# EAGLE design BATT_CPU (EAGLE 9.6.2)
COMPANY: ADAFRUIT INDUSTRIES; DRAWN: KTOWN; REV: B
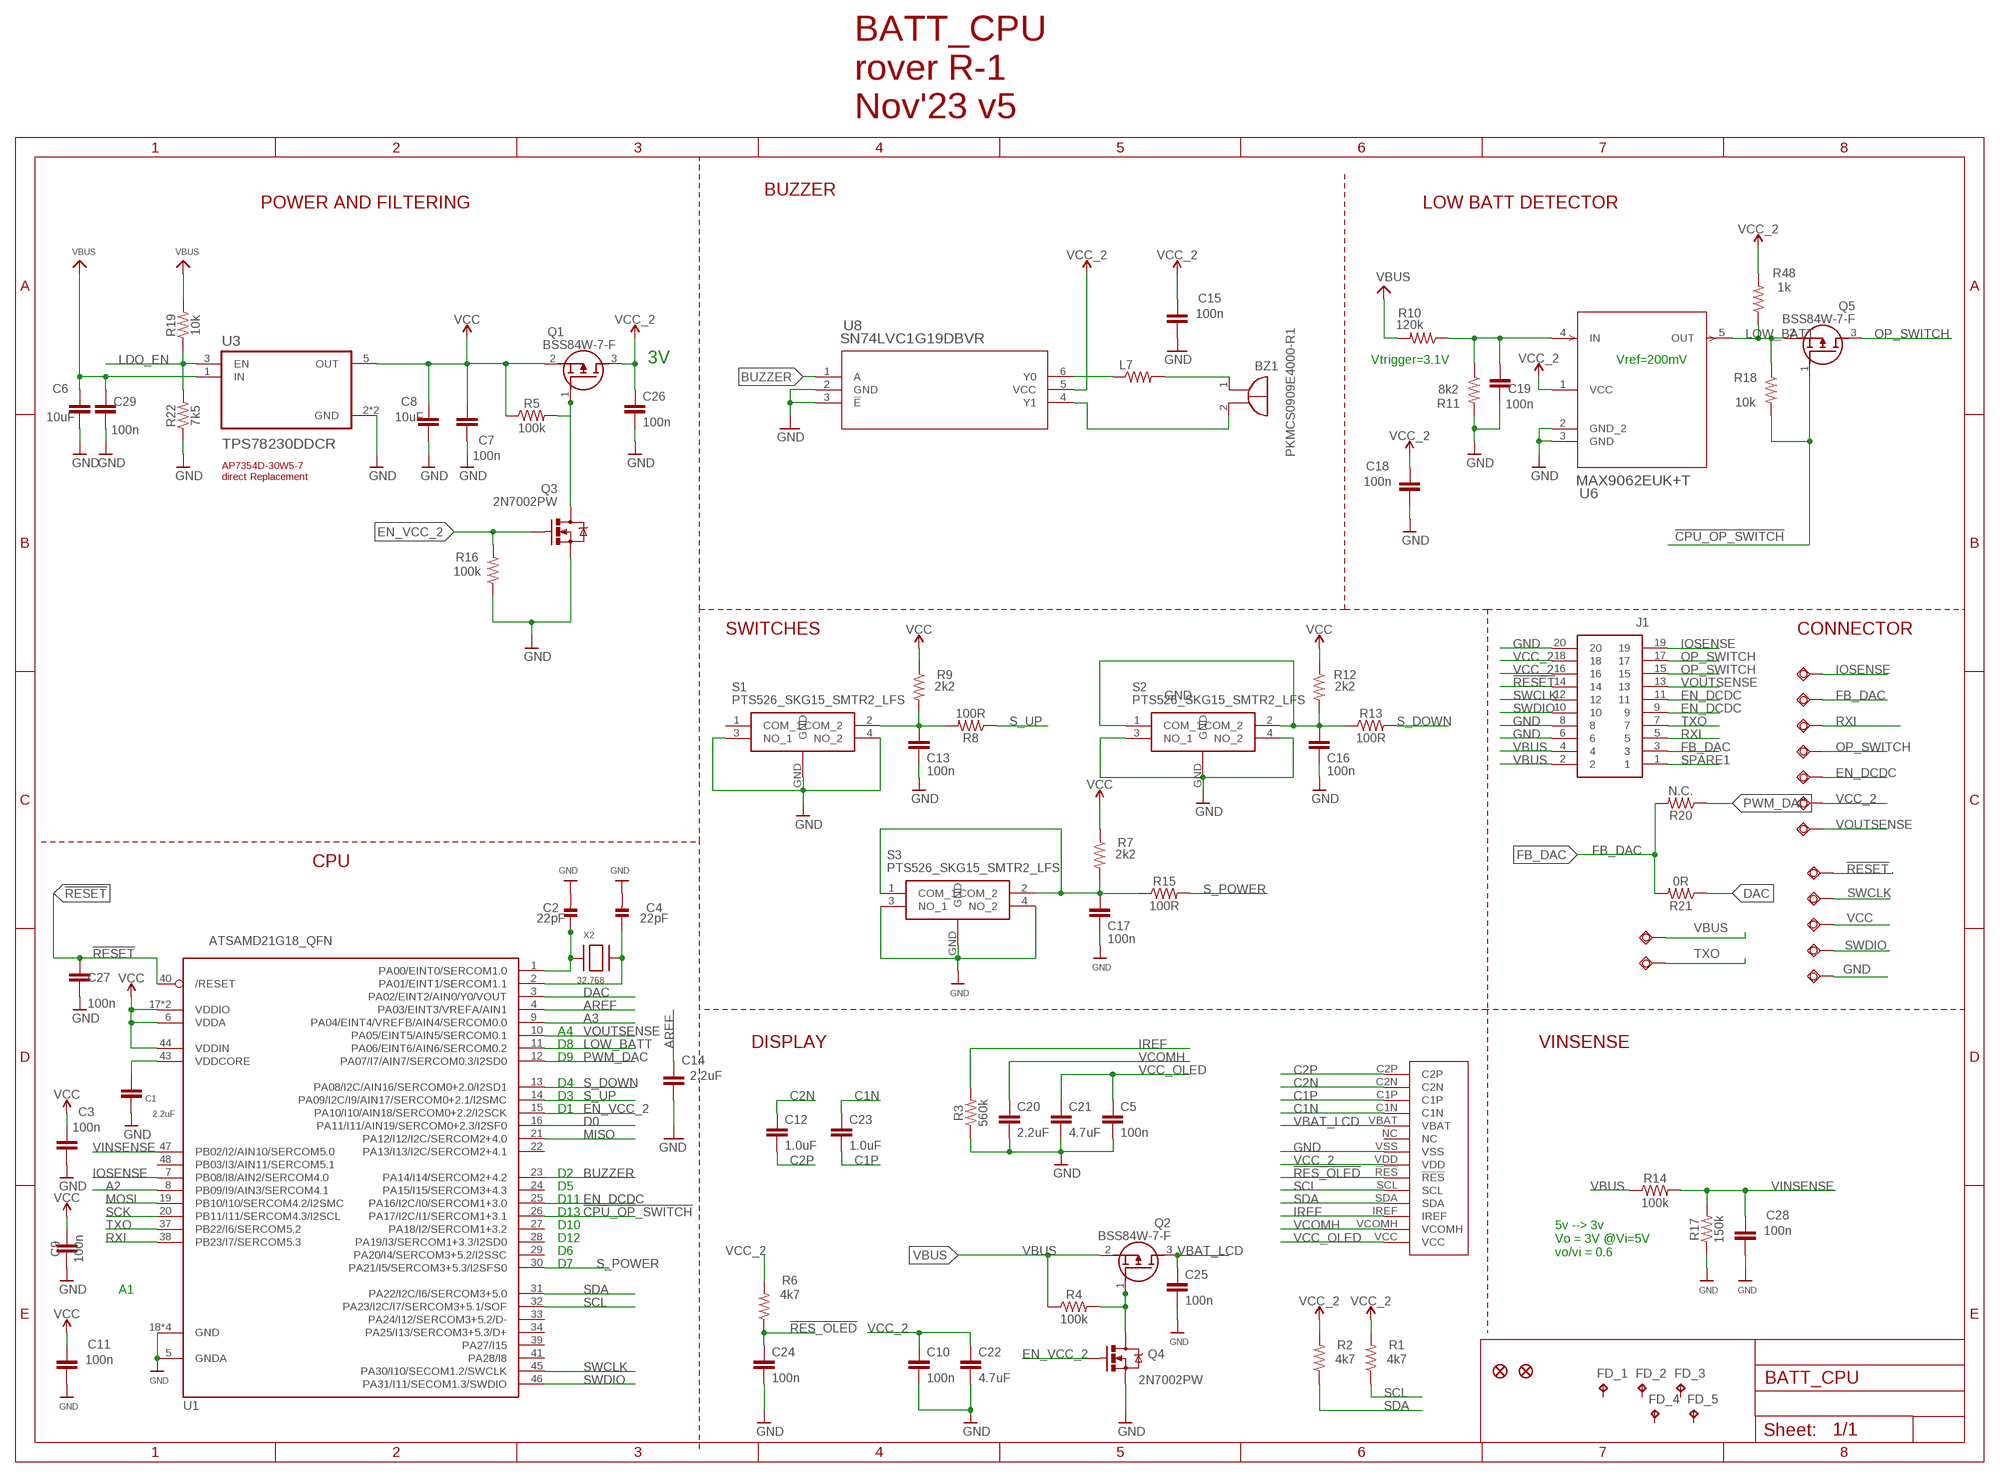
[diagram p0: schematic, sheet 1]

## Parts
BZ1  PKMCS0909E4000-R1  [PKMCS0909]
C1  2.2uF  2.2UF-0603-10V-20%  [0603]
C2  22pF  CAP_CERAMIC0603_NO  [0603-NO]
C3  100n  0.1UF-0402-16V-10%  [0402]
C4  22pF  CAP_CERAMIC0603_NO  [0603-NO]
C5  100n  0.1UF-0402-16V-10%  [0402]
C6  10uF  2.2UF-0603-10V-20%  [0603]
C7  100n  0.1UF-0402-16V-10%  [0402]
C8  10uF  2.2UF-0603-10V-20%  [0603]
C9  100n  0.1UF-0402-16V-10%  [0402]
C10  100n  0.1UF-0402-16V-10%  [0402]
C11  100n  0.1UF-0402-16V-10%  [0402]
C12  1.0uF  1.0UF-0402-16V-10%  [0402]
C13  100n  0.1UF-0402-16V-10%  [0402]
C14  2.2uF  2.2UF-0603-10V-20%  [0603]
C15  100n  0.1UF-0402-16V-10%  [0402]
C16  100n  0.1UF-0402-16V-10%  [0402]
C17  100n  0.1UF-0402-16V-10%  [0402]
C18  100n  0.1UF-0402-16V-10%  [0402]
C19  100n  0.1UF-0402-16V-10%  [0402]
C20  2.2uF  2.2UF-0603-10V-20%  [0603]
C21  4.7uF  4.7UF0603  [0603]
C22  4.7uF  4.7UF0603  [0603]
C23  1.0uF  1.0UF-0402-16V-10%  [0402]
C24  100n  0.1UF-0402-16V-10%  [0402]
C25  100n  0.1UF-0402-16V-10%  [0402]
C26  100n  0.1UF-0402-16V-10%  [0402]
C27  100n  0.1UF-0402-16V-10%  [0402]
C28  100n  0.1UF-0402-16V-10%  [0402]
C29  100n  0.1UF-0402-16V-10%  [0402]
EN_DCDC  TESTPAD_TPSQB1,27  [TESTPAD_B1,27]
FB_DAC  TESTPAD_TPSQB1,27  [TESTPAD_B1,27]
FD_1  FD_1  TPTP06SQ  [TP06SQ]
FD_2  FD_1  TPTP06SQ  [TP06SQ]
FD_3  FD_1  TPTP06SQ  [TP06SQ]
FD_4  FD_1  TPTP06SQ  [TP06SQ]
FD_5  FD_1  TPTP06SQ  [TP06SQ]
IOSENSE  TESTPAD_TPSQB1,27  [TESTPAD_B1,27]
J1  DF40C_2.0_-20DS-0.4V_51_  [DF40C2020DS04V51]
L7  MMZ2012Y202BT000  RESISTOR0805-RES  [0805]
OP_SWITCH  TESTPAD_TPSQB1,27  [TESTPAD_B1,27]
Q1  BSS84W-7-F  [SOT65P222X110-3N]
Q2  BSS84W-7-F  [SOT65P222X110-3N]
Q3  2N7002PW  MOSFET-NCHANNEL2N7002PW  [SOT323]
Q4  2N7002PW  MOSFET-NCHANNEL2N7002PW  [SOT323]
Q5  BSS84W-7-F  [SOT65P222X110-3N]
R1  4k7  RESISTOR0402  [0402]
R2  4k7  RESISTOR0402  [0402]
R3  560k  RESISTOR0402  [0402]
R4  100k  RESISTOR0402  [0402]
R5  100k  RESISTOR0402  [0402]
R6  4k7  RESISTOR0402  [0402]
R7  2k2  RESISTOR0402  [0402]
R8  100R  RESISTOR0402  [0402]
R9  2k2  RESISTOR0402  [0402]
R10  120k  RESISTOR0402  [0402]
R11  8k2  RESISTOR0402  [0402]
R12  2k2  RESISTOR0402  [0402]
R13  100R  RESISTOR0402  [0402]
R14  100k  RESISTOR0402  [0402]
R15  100R  RESISTOR0402  [0402]
R16  100k  RESISTOR0402  [0402]
R17  150k  RESISTOR0402  [0402]
R18  10k  RESISTOR0402  [0402]
R19  10k  RESISTOR0402  [0402]
R20  N.C.  RESISTOR0402  [0402]
R21  0R  RESISTOR0402  [0402]
R22  7k5  RESISTOR0402  [0402]
R48  1k  RESISTOR0402  [0402]
RXI  TESTPAD_TPSQB1,27  [TESTPAD_B1,27]
S1  PTS526_SKG15_SMTR2_LFS  [PTS526SKG15SMTR2LFS]
S2  PTS526_SKG15_SMTR2_LFS  [PTS526SKG15SMTR2LFS]
S3  PTS526_SKG15_SMTR2_LFS  [PTS526SKG15SMTR2LFS]
U1  ATSAMD21G18_QFN  ATSAMD21J_QFN  [TQFN48_7MM]
U3  TPS78230DDCR  [SOT95P280X110-5N]
U6  MAX9062EUK+T  [21-0057F_MXM]
U8  SN74LVC1G19DBVR  [DBV6]
U$30  64X32_OLED_049  [LCD_14_PINS]
U$34  FIDUCIAL""  [FIDUCIAL_1MM]
U$35  FIDUCIAL""  [FIDUCIAL_1MM]
VBUS  TESTPAD_TPSQB1,27  [TESTPAD_B1,27]
VBUS1  TESTPAD_TPSQB1,27  [TESTPAD_B1,27]
VBUS2  TESTPAD_TPSQB1,27  [TESTPAD_B1,27]
VBUS3  TESTPAD_TPSQB1,27  [TESTPAD_B1,27]
VBUS4  TESTPAD_TPSQB1,27  [TESTPAD_B1,27]
VBUS5  TESTPAD_TPSQB1,27  [TESTPAD_B1,27]
VBUS6  TESTPAD_TPSQB1,27  [TESTPAD_B1,27]
VCC_2  TESTPAD_TPSQB1,27  [TESTPAD_B1,27]
VOUTSENSE  TESTPAD_TPSQB1,27  [TESTPAD_B1,27]
X2  32.768  XTAL-3.2X1.5  [XTAL3215]

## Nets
!CPU_OP_SWITCH: Q5.1(G) R18.2 U1.26(PA17/I2C/I1/SERCOM1+3.1)
!RES_OLED: C24.1 R6.1 U$30.!RES
!RESET: C27.1 J1.14 U1.40(/RESET) VBUS1.TP
A2: U1.8(PB09/I9/AIN3/SERCOM4.1)
A3: U1.9(PA04/EINT4/VREFB/AIN4/SERCOM0.0)
AREF: C14.1 U1.4(PA03/EINT3/VREFA/AIN1)
BUZZER: U1.23(PA14/I14/SERCOM2+4.2) U8.1(A)
C1N: C23.1 U$30.C1N
C1P: C23.2 U$30.C1P
C2N: C12.1 U$30.C2N
C2P: C12.2 U$30.C2P
D0: U1.16(PA11/I11/AIN19/SERCOM0+2.3/I2SF0)
DAC: R21.1 U1.3(PA02/EINT2/AIN0/Y0/VOUT)
EN_DCDC: EN_DCDC.TP J1.9 J1.11 U1.25(PA16/I2C/I0/SERCOM1+3.0)
EN_VCC_2: Q3.1(G) Q4.1(G) R16.2 U1.15(PA10/I10/AIN18/SERCOM0+2.2/I2SCK)
FB_DAC: FB_DAC.TP J1.3 R20.2 R21.2
GND: C1.2 C2.2 C3.2 C4.2 C5.2 C6.2 C7.2 C8.2 C9.2 C10.2 C11.2 C13.2 C14.2 C15.2 C16.2 C17.2 C18.2 C19.2 C20.2 C21.2 C22.2 C24.2 C25.2 C26.2 C27.2 C28.2 C29.2 J1.6 J1.8 J1.20 Q3.2(S) Q4.2(S) R3.1 R11.2 R16.1 R17.1 R22.1 S1.3(NO_1) S1.4(NO_2) S1.GND S2.3(NO_1) S2.4(NO_2) S2.GND S3.3(NO_1) S3.4(NO_2) S3.GND U1.5(GNDA) U1.18(GND) U1.35(GND) U1.42(GND) U1.THERMAL(GND) U3.2(GND) U3.4(GND) U6.2(GND_2) U6.3(GND) U8.2(GND) U8.3(!E) U$30.VSS VBUS4.TP
IOSENSE: IOSENSE.TP J1.19 U1.7(PB08/I8/AIN2/SERCOM4.0)
IREF: R3.2 U$30.IREF
LDO_EN: R19.1 R22.2 U3.3(EN)
LOW_BATT: Q5.2(S) R18.1 R48.1 U1.11(PA06/EINT6/AIN6/SERCOM0.2) U6.5(OUT)
MISO: U1.21(PA12/I12/I2C/SERCOM2+4.0)
MOSI: U1.19(PB10/I10/SERCOM4.2/I2SMC)
N$1: C17.1 R7.2 R15.1 S3.1(COM_1) S3.2(COM_2)
N$2: C13.1 R8.2 R9.2 S1.2(COM_2)
N$3: C16.1 R12.2 R13.1 S2.1(COM_1) S2.2(COM_2)
N$4: Q2.1(G) Q4.3(D) R4.2
N$5: C2.1 U1.1(PA00/EINT0/SERCOM1.0) X2.P$1
N$6: Q1.1(G) Q3.3(D) R5.2
N$7: C4.1 U1.2(PA01/EINT1/SERCOM1.1) X2.P$2
N$10: C19.1 R10.1 R11.1 U6.4(IN)
N$17: L7.1 U8.6(Y0)
N$19: BZ1.1(+) L7.2
N$22: BZ1.2(-) U8.4(Y1)
OP_SWITCH: J1.15 J1.17 OP_SWITCH.TP Q5.3(D)
PWM_DAC: R20.1 U1.12(PA07/I7/AIN7/SERCOM0.3/I2SD0)
RXI: J1.5 RXI.TP U1.38(PB23/I7/SERCOM5.3)
S_DOWN: R13.2 U1.13(PA08/I2C/AIN16/SERCOM0+2.0/I2SD1)
S_POWER: R15.2 U1.30(PA21/I5/SERCOM3+5.3/I2SFS0)
S_UP: R8.1 U1.14(PA09/I2C/I9/AIN17/SERCOM0+2.1/I2SMC)
SCK: U1.20(PB11/I11/SERCOM4.3/I2SCL)
SCL: R1.1 U1.32(PA23/I2C/I7/SERCOM3+5.1/SOF) U$30.SCL
SDA: R2.1 U1.31(PA22/I2C/I6/SERCOM3+5.0) U$30.SDA
SPARE1: J1.1
SWCLK: J1.12 U1.45(PA30/I10/SECOM1.2/SWCLK) VBUS2.TP
SWDIO: J1.10 U1.46(PA31/I11/SECOM1.3/SWDIO) VBUS3.TP
TXO: J1.7 U1.37(PB22/I6/SERCOM5.2) VBUS6.TP
VBAT_LCD: C25.1 Q2.3(D) U$30.VBAT
VBUS: C6.1 C29.1 J1.2 J1.4 Q2.2(S) R4.1 R10.2 R14.1 R19.2 U3.1(IN) VBUS5.TP
VCC: C3.1 C7.1 C8.1 C9.1 C11.1 Q1.2(S) R5.1 R7.1 R9.1 R12.1 R48.2 U1.6(VDDA) U1.17(VDDIO) U1.36(VDDIO) U1.44(VDDIN) U3.5(OUT) VBUS.TP ; supply symbol labelled VCC_2
VCC_2: C10.1 C15.1 C18.1 C22.1 C26.1 J1.16 J1.18 Q1.3(D) R1.2 R2.2 R6.2 U6.1(VCC) U8.5(VCC) U$30.VDD VCC_2.TP
VCC_OLED: C5.1 C21.1 U$30.VCC
VCOMH: C20.1 U$30.VCOMH
VDDCORE: C1.1 U1.43(VDDCORE)
VINSENSE: C28.1 R14.2 R17.2 U1.47(PB02/I2/AIN10/SERCOM5.0)
VOUTSENSE: J1.13 U1.10(PA05/EINT5/AIN5/SERCOM0.1) VOUTSENSE.TP
Unconnected: FD_1.TP FD_2.TP FD_3.TP FD_4.TP FD_5.TP S1.1(COM_1) U1.22(PA13/I13/I2C/SERCOM2+4.1) U1.24(PA15/I15/SERCOM3+4.3) U1.27(PA18/I2/SERCOM1+3.2) U1.28(PA19/I3/SERCOM1+3.3/I2SD0) U1.29(PA20/I4/SERCOM3+5.2/I2SSC) U1.33(PA24/I12/SERCOM3+5.2/D-) U1.34(PA25/I13/SERCOM3+5.3/D+) U1.39(PA27/I15) U1.41(PA28/I8) U1.48(PB03/I3/AIN11/SERCOM5.1) U$30.NC

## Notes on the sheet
- BATT_CPU
  rover R-1
  Nov'23 v5
- BUZZER
- POWER AND FILTERING | LOW BATT DETECTOR
- 3V | Vtrigger=3.1V | Vref=200mV
- AP7354D-30W5-7 
  direct Replacement
- SWITCHES | CONNECTOR
- CPU
- A4
- D8 | DISPLAY | VINSENSE
- D9
- D4
- D3
- D1
- D2
- D5
- D11
- D13
- D10
- D12
- D6
- D7
- 5v --> 3v
  Vo = 3V @Vi=5V
  vo/vi = 0.6
- A1

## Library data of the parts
BZ1 = buzzer:PKMCS0909E4000-R1: PKMCS0909E4000-R1
C1 C14 C20 = SparkFun-Capacitors:2.2UF: 2.2µF ceramic capacitors; PROD_ID: CAP-07888
C2 C4 = microbuilder:CAP_CERAMIC: Ceramic Capacitors
C3 C5 C7 C9-C11 C13 C15-C19 C24-C29 = SparkFun-Capacitors:0.1UF: 0.1µF ceramic capacitors; PROD_ID: CAP-12416; VALUE: 0.1uF
C6 C8 = SparkFun-Capacitors:2.2UF: 2.2µF ceramic capacitors; PROD_ID: CAP-07888; VALUE: 2.2uF
C12 C23 = SparkFun-Capacitors:1.0UF: 1µF ceramic capacitors; PROD_ID: CAP-12417
C21 C22 = SparkFun-Capacitors:4.7UF: 4.7µF ceramic capacitors; PROD_ID: CAP-08280
EN_DCDC FB_DAC IOSENSE OP_SWITCH RXI VBUS VBUS1-VBUS6 VCC_2 VOUTSENSE = BeagleBone_Blue_R3:TESTPAD_TPSQ: Test pad
FD_1-FD_5 = testpad:TP: Test pad
J1 = DF40C_2.0_-20DS-0.4V_51_:DF40C_2.0_-20DS-0.4V_51_: Board to Board & Mezzanine Connectors 20P 2-ROW RECEPT VERT SMT 2.0MM HGHT Source: Datasheet; DESCRIPTION: Board to Board & Mezzanine Connectors 20P 2-ROW RECEPT VERT SMT 2.0MM HGHT; HEIGHT: 2.1mm; MANUFACTURER_NAME: Hirose; MANUFACTURER_PART_NUMBER: DF40C(2.0)-20DS-0.4V(51); MOUSER_PART_NUMBER: 798-DF40C2020DS04V51; MOUSER_PRICE-STOCK: https://www.mouser.co.uk/ProductDetail/Hirose-Connector/DF40C2.0-20DS-0.4V51?qs=3aug5cyrIbdA5dYbMRd5pw%3D%3D
L7 = SparkFun:RESISTOR: Resistor
Q1 Q2 Q5 = BSS84W-7-F:BSS84W-7-F: Lattice Source: Datasheet; DESCRIPTION: Lattice; HEIGHT: 1.1mm; MANUFACTURER_NAME: Lattice Semiconductor; MANUFACTURER_PART_NUMBER: BSS84W-7-F; MOUSER_PART_NUMBER: N/A; MOUSER_PRICE-STOCK: https://www.mouser.com/Search/Refine.aspx?Keyword=N%2FA
Q3 Q4 = SparkFun-DiscreteSemi:MOSFET-NCHANNEL: Common NMOSFET Parts MFG P/NStore IDProd ID FDD8780TRANS-09984 SI7820DNTRANS-11055 FDS6630AIC-08089 2N7002PWTRANS-11151 FQP30N06L COM-10213TRANS-10060 BSS123LT1GTRANS-08345 BSS138TRANS-00830 BS170 2N7000; PROD_ID: TRANS-11151
R1-R22 R48 = SparkFun-Resistors:RESISTOR: Generic Resistor Package
S1-S3 = PTS526_SKG15_SMTR2_LFS:PTS526_SKG15_SMTR2_LFS: Tact 5.2 x 5.2, 1.5 mm H, 260gf, G leads, Ground pin, metal actuator Source: Datasheet; ARROW_PART_NUMBER: PTS526 SKG15 SMTR2 LFS; ARROW_PRICE-STOCK: https://www.arrow.com/en/products/pts526-skg15-smtr2-lfs/ck?region=nac; DESCRIPTION: Tact 5.2 x 5.2, 1.5 mm H, 260gf, G leads, Ground pin, metal actuator; HEIGHT: 1.6mm; MANUFACTURER_NAME: C & K COMPONENTS; MANUFACTURER_PART_NUMBER: PTS526 SKG15 SMTR2 LFS; MOUSER_PART_NUMBER: 611-PTS526SKG15SMR2L; MOUSER_PRICE-STOCK: https://www.mouser.co.uk/ProductDetail/CK/PTS526-SKG15-SMTR2-LFS?qs=UXgszm6BlbEc7nn5s4cd2Q%3D%3D
U1 = microbuilder:ATSAMD21J
U3 = TPS78230DDCR:TPS78230DDCR: Check prices; AVAILABILITY: Good; DESCRIPTION: 150-mA, nano-IQ, low-dropout voltage regulator with enable from -40C to +125C 5-SOT-23-THIN -40 to 125; MF: Texas Instruments; MP: TPS78230DDCR; PACKAGE: SOT-23-THN-5 Texas Instruments; PRICE: None; PURCHASE-URL: https://pricing.snapeda.com/search/part/TPS78230DDCR/?ref=eda
U6 = MAX9062:MAX9062EUK+T; BUILT_BY: EMA_UL_Team; MANUFACTURER_PART_NUMBER: MAX9062EUK+T; SOURCELIBRARY: Maxim_2014-06-20; VENDOR: Maxim Integrated Products
U8 = SN74LVC1G19DBVR:SN74LVC1G19DBVR; DATASHEET_URL: http://www.ti.com/lit/gpn/SN74LVC1G19; DESCRIPTION: 1-of-2 Decoder/Demultiplexer; FAMILY_NAME: LL Decoder, Mux/Demux; GENERIC_PART_NUMBER: SN74LVC1G19; INDUSTRY_STD_PKG_TYPE: SOT-23; MANUFACTURER: Texas Instruments; MANUFACTURER_PART_NUMBER: SN74LVC1G19DBVR; PACKAGE_DESIGNATOR: DBV; PIN_COUNT: 6; VENDOR: Texas Instruments
U$30 = OLED 66 64x48:64X32_OLED_049
U$34 U$35 = microbuilder:FIDUCIAL: Fiducial Alignment Points; BOM: EXCLUDE
X2 = adafruit2:XTAL: Low cost SMT crystals, no capacitors included

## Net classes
2 gnd: width 0.305 mm, drill 0.483 mm, clearance 0.203 mm

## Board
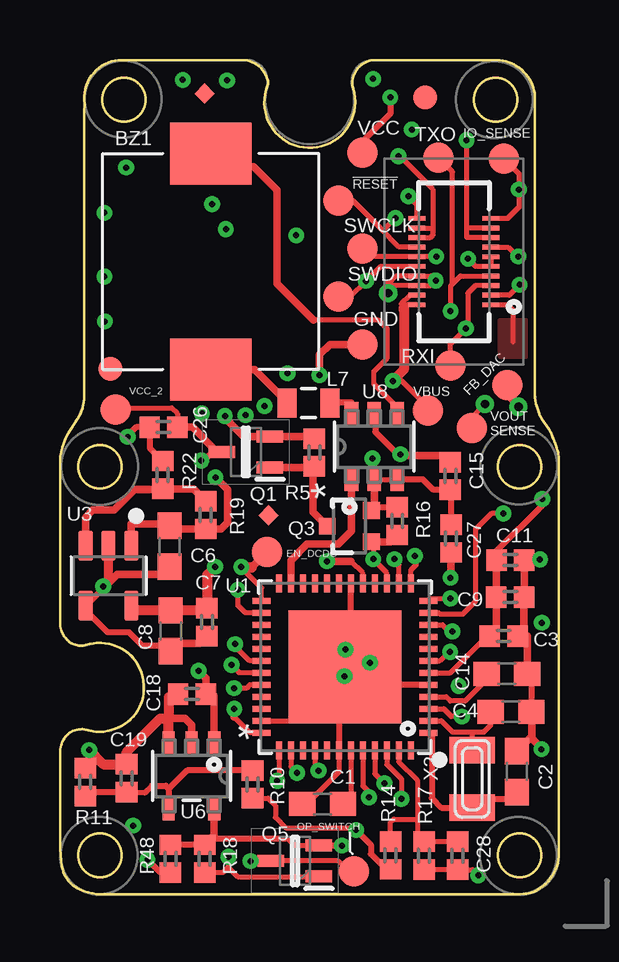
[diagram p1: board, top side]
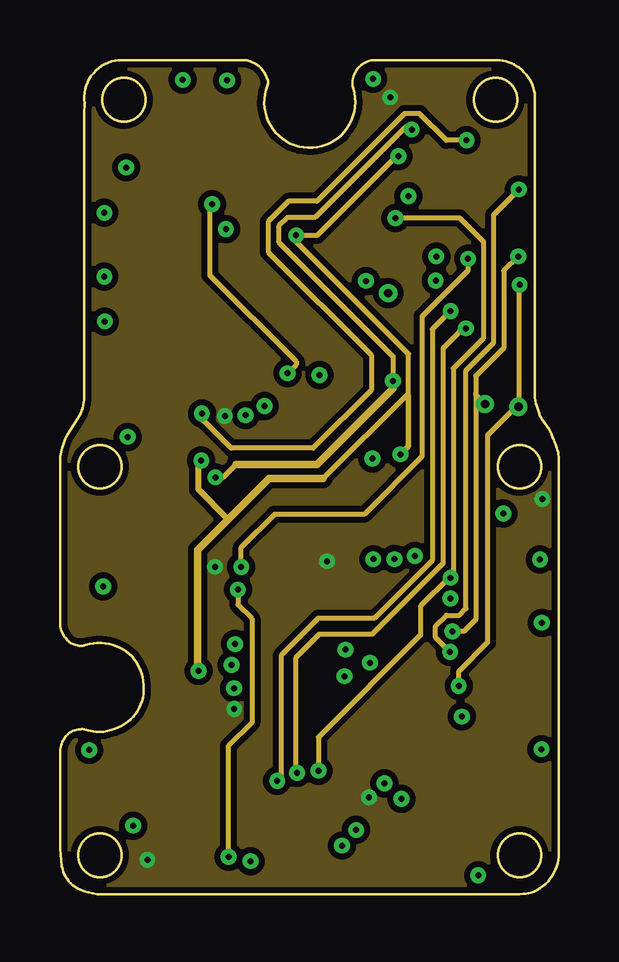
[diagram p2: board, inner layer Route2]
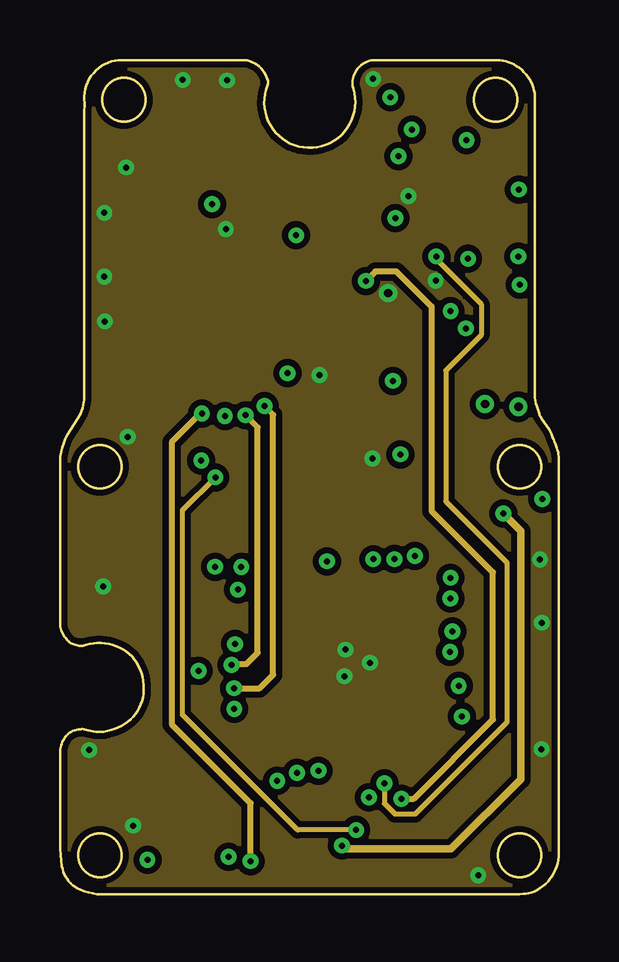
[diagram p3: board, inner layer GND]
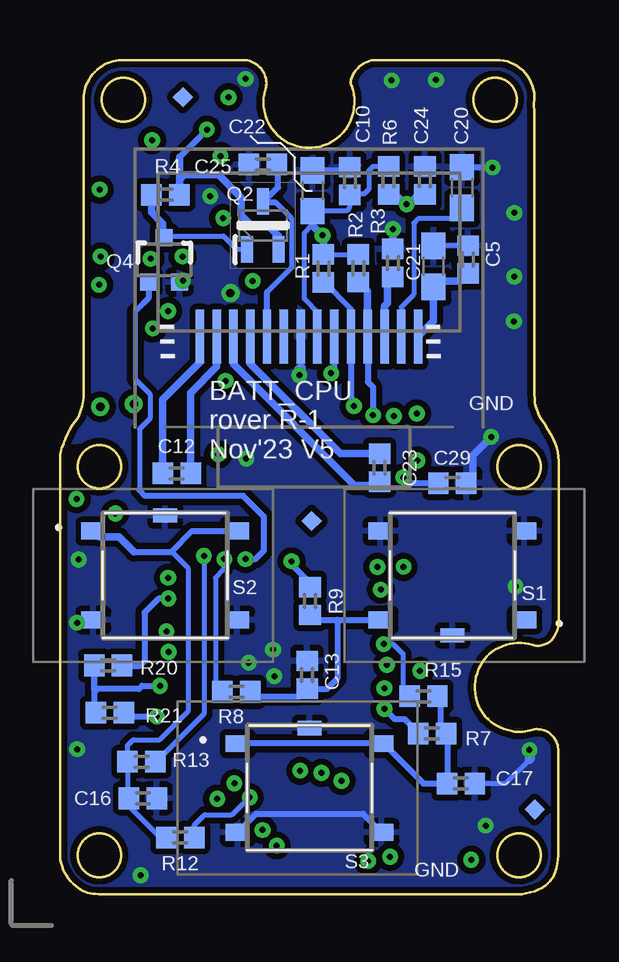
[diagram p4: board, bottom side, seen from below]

Size 20.8 x 34.78 mm. Coordinates in mm from the lower left corner, seen from the top.
Outline: 7.81,34.77 2.6,34.78 arc99 1.03,32.97 1.02,32.57 1.02,21.34 arc-3 1,20.62 arc-31 0.74,19.84 arc4 0.31,19.14 arc31 0,17.87 0,11.35 arc48 0.36,10.55 arc58 1.08,10.39 arc-37 2.36,10.34 arc-41 3.27,9.53 arc-39 3.46,8.21 arc-46 2.7,7.1 arc-24 1.83,6.78 arc-26 1.18,6.84 arc65 0.27,6.61 arc38 0.02,6.05 0.02,1.89 arc10 0.08,1.17 arc56 0.83,0.2 arc27 1.92,0 18.85,0 arc2 19.32,0.01 arc33 20.04,0.26 arc26 20.6,0.9 arc24 20.8,1.58 20.8,18.16 arc21 20.72,18.6 arc-1 20.65,18.79 arc1 20.56,19.03 arc19 20.09,19.82 arc-27 19.98,20.04 arc9 19.92,20.23 arc-24 19.81,20.83 19.81,33.17 arc26 19.65,33.85 arc31 19.04,34.53 arc31 18.22,34.78 13.18,34.78 arc83 12.2,33.91 arc24 12.23,33.58 arc-219 8.65,33.72 arc39 8.66,33.96 arc59 7.81,34.77
Outline: circle at 18.16,33.13 radius 0.9
Outline: circle at 19.16,17.83 radius 0.9
Outline: circle at 19.16,1.63 radius 0.9
Outline: circle at 1.66,1.63 radius 0.9
Outline: circle at 1.66,17.83 radius 0.9
Outline: circle at 2.66,33.13 radius 0.9
Copper layers (1+2*15+16): Top 0.035mm / dielectric 1.5mm / Route2 0.035mm / dielectric 0.15mm / GND 0.035mm / dielectric 0.2mm / Bottom 0.035mm
Design rules "adafruit *": minimum track width 8mil, minimum drill 0.25mm, track to track 8mil, track to pad 8mil, pad to pad 8mil, via to via 8mil, smd to smd 5mil, copper to edge 10mil, drill to drill 8mil, minimum pad ring 10mil, minimum via ring 8mil, stop-mask expansion 2mil, vias tented up to drill 20mil, thermal gap 10mil
bRestrict: area 20,17.1 to 20.7,18.5

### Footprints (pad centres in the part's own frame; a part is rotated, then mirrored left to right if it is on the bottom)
PKMCS0909 = smd 2.6 x 3.4: 1 -4.5,0; 2 4.5,0
0603 = smd 1.1 x 1: 1 -0.85,0; 2 0.85,0
0603-NO = smd 1.1 x 1: 1 -0.85,0; 2 0.85,0
0402 = smd 0.85 x 0.9: 1 -0.58,0; 2 0.58,0
TESTPAD_B1,27 = smd 1.27 x 1.27: TP 0,0
TP06SQ = smd 0.6 x 0.6: TP 0,0
DF40C2020DS04V51 = smd 0.2 x 0.7: 1 -1.8,-1.54; 2 -1.8,1.54; 3 -1.4,-1.54; 4 -1.4,1.54; 5 -1,-1.54; 6 -1,1.54; 7 -0.6,-1.54; 8 -0.6,1.54; 9 -0.2,-1.54; 10 -0.2,1.54; 11 0.2,-1.54; 12 0.2,1.54; 13 0.6,-1.54; 14 0.6,1.54; 15 1,-1.54; 16 1,1.54; 17 1.4,-1.54; 18 1.4,1.54; 19 1.8,-1.54; 20 1.8,1.54
0805 = smd 0.8 x 1.2: 1 -0.9,0; 2 0.9,0
SOT65P222X110-3N = smd 1.1 x 0.5: 1 -1,0.65; 2 -1,-0.65; 3 1,0
SOT323 = smd 0.7 x 0.7: 1 -0.65,-0.925; 2 0.65,-0.925; 3 0,0.925
PTS526SKG15SMTR2LFS = smd 1 x 0.7: 1 -3,1.85; 2 3,1.85; 3 -3,-1.85; 4 3,-1.85 | smd 1 x 0.6: GND 0,2.5
TQFN48_7MM = smd 0.25 x 0.75: 1 -2.75,-3.475; 2 -2.25,-3.475; 3 -1.75,-3.475; 4 -1.25,-3.475; 5 -0.75,-3.475; 6 -0.25,-3.475; 7 0.25,-3.475; 8 0.75,-3.475; 9 1.25,-3.475; 10 1.75,-3.475; 11 2.25,-3.475; 12 2.75,-3.475; 25 2.75,3.475; 26 2.25,3.475; 27 1.75,3.475; 28 1.25,3.475; 29 0.75,3.475; 30 0.25,3.475; 31 -0.25,3.475; 32 -0.75,3.475; 33 -1.25,3.475; 34 -1.75,3.475; 35 -2.25,3.475; 36 -2.75,3.475 | smd 0.75 x 0.25: 13 3.475,-2.75; 14 3.475,-2.25; 15 3.475,-1.75; 16 3.475,-1.25; 17 3.475,-0.75; 18 3.475,-0.25; 19 3.475,0.25; 20 3.475,0.75; 21 3.475,1.25; 22 3.475,1.75; 23 3.475,2.25; 24 3.475,2.75; 37 -3.475,2.75; 38 -3.475,2.25; 39 -3.475,1.75; 40 -3.475,1.25; 41 -3.475,0.75; 42 -3.475,0.25; 43 -3.475,-0.25; 44 -3.475,-0.75; 45 -3.475,-1.25; 46 -3.475,-1.75; 47 -3.475,-2.25; 48 -3.475,-2.75 | smd 4.7 x 4.7: THERMAL 0,0
SOT95P280X110-5N = smd 1.25 x 0.59: 1 -1.255,0.95; 2 -1.255,0; 3 -1.255,-0.95; 4 1.255,-0.95; 5 1.255,0.95
21-0057F_MXM = smd 0.972 x 0.508: 1 -1.362,0.95; 2 -1.362,0; 3 -1.362,-0.95; 4 1.362,-0.95; 5 1.362,0.95
DBV6 = smd 0.972 x 0.568: 1 -1.362,0.95; 2 -1.362,0; 3 -1.362,-0.95; 4 1.362,-0.95; 5 1.362,0; 6 1.362,0.95
LCD_14_PINS = smd 0.35 x 2.25: !RES 5.6,1.125; C1N 2.1,1.125; C1P 1.4,1.125; C2N 0.7,1.125; C2P 0,1.125; IREF 7.7,1.125; NC 3.5,1.125; SCL 6.3,1.125; SDA 7,1.125; VBAT 2.8,1.125; VCC 9.1,1.125; VCOMH 8.4,1.125; VDD 4.9,1.125; VSS 4.2,1.125
FIDUCIAL_1MM = smd 1 x 1: 1 0,0
XTAL3215 = smd 1.1 x 1.9: P$1 1.2,0; P$2 -1.2,0

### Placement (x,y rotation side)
BZ1  6.29,26.38 90 top
C1  10.95,3.77 180 top
C2  19.06,5.12 90 top
C3  18.5,10.77 0 top
C4  18.81,7.61 0 top
C5  3.78,26.46 90 bottom
C6  4.57,14.51 270 top
C7  6.13,11.35 270 top
C8  4.61,10.99 270 top
C9  18.77,12.39 0 top
C10  8.71,29.73 90 bottom
C11  18.78,13.93 0 top
C12  15.93,17.55 180 bottom
C13  10.49,9.15 90 bottom
C14  18.64,9.2 0 top
C15  16.27,17.44 270 top
C16  17.34,4 0 bottom
C17  4.08,4.62 0 bottom
C18  5.51,8.35 180 top
C19  2.78,4.84 90 top
C20  4.03,29.46 90 bottom
C21  5.22,26.18 90 bottom
C22  10.26,29.33 90 bottom
C23  7.47,17.78 270 bottom
C24  5.58,29.76 90 bottom
C25  12.34,30.42 180 bottom
C26  4.32,19.47 180 top
C27  16.31,14.83 90 top
C28  16.58,1.61 270 top
C29  4.44,17.14 0 bottom
EN_DCDC  8.63,14.26 0 top
FB_DAC  18.66,21.22 0 top
FD_1  15.67,33.23 45 bottom
FD_2  1,3.53 45 bottom
FD_3  10.31,15.57 45 bottom
FD_4  6.03,33.38 135 top
FD_5  8.7,15.8 45 top
IOSENSE  18.52,30.67 0 top
J1  16.43,26.38 90 top
L7  10.37,20.48 180 top
OP_SWITCH  12.27,0.96 0 top
Q1  7.75,18.45 180 top
Q2  12.34,27.88 90 bottom
Q3  12.07,15.35 90 top
Q4  16.46,26.45 0 bottom
Q5  9.8,1.39 180 top
R1  9.82,26.09 90 bottom
R2  8.36,26.1 90 bottom
R3  6.92,26.32 270 bottom
R4  16.4,29.16 180 bottom
R5  10.61,18.42 270 top
R6  7.1,29.76 90 bottom
R7  5.28,6.7 0 bottom
R8  13.45,8.44 0 bottom
R9  10.37,12.23 270 bottom
R10  8.03,4.59 270 top
R11  1.06,4.68 90 top
R12  15.78,2.37 180 bottom
R13  17.4,5.53 0 bottom
R14  13.79,1.62 90 top
R15  5.64,8.26 180 bottom
R16  14.06,15.56 270 top
R17  15.18,1.61 90 top
R18  6.04,1.48 270 top
R19  6.08,15.81 270 top
R20  18.79,9.54 180 bottom
R21  18.72,7.57 180 bottom
R22  4.29,17.48 270 top
R48  4.61,1.49 270 top
RXI  16.28,22.05 0 top
S1  4.43,13.29 180 bottom
S2  16.41,13.29 0 bottom
S3  10.39,4.44 0 bottom
U1  11.88,9.48 90 top
U3  2.02,13.29 270 top
U6  5.49,4.94 270 top
U8  13.11,18.66 90 top
U$30  14.96,22.12 0 bottom
U$34  15.23,33.21 0 top
U$35  2.11,21.92 0 top
VBUS  12.61,30.91 0 top
VBUS1  11.61,28.91 0 top
VBUS2  12.61,26.91 0 top
VBUS3  11.61,24.91 0 top
VBUS4  12.61,22.92 0 top
VBUS5  15.35,20.17 0 top
VBUS6  15.78,30.71 0 top
VCC_2  2.32,20.21 0 top
VOUTSENSE  17.17,19.43 0 top
X2  17.2,4.81 270 top

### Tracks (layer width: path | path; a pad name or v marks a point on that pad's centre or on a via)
!CPU_OP_SWITCH  (via drill 0.25)
  Top 0.203: U1.26 7.73,11.73 7.42,12.04 v7.42,12.7 | R18.2 6.79,0.9 7.03,1.14 v7.03,1.56 7.03,1.11 7.43,0.71 10.77,0.71 Q5.1
  Route2 0.203: v7.03,1.56 7.03,6.18 8,7.15 8,11.49 7.42,12.07 v7.42,12.7
!RES_OLED  (via drill 0.25)
  Route2 0.203: v9.49,21.72 9.86,22.09 9.86,22.2 6.24,25.82 6.24,28.68 v6.34,28.78
  Bottom 0.203: C24.1 5.94,29.18 v6.34,28.78 6.75,29.18 R6.1
  Bottom 0.254: U$30.!RES 9.36,21.85 v9.49,21.72
!RESET  (via drill 0.25)
  Top 0.203: v10.78,5.16 10.63,5.31 U1.40 | J1.14 14.14,26.99 13.41,27.72 | VBUS1.TP 12.22,28.91 13.41,27.72 | 13.41,27.72 13.52,27.72 v13.99,28.19
  Top 0.305: C27.1 16.31,13.22 v16.29,13.2
  Route2 0.203: v10.78,5.16 10.78,6.55 15.04,10.81 15.04,12.02 16.22,13.2 v16.29,13.2 16.4,13.31 16.4,21.92 17.67,23.19 17.67,27.19 16.67,28.19 v13.99,28.19
AREF
  Top 0.203: C14.1 17.79,8.94 16.9,8.05 16.28,8.05 16.1,8.23 U1.4
BUZZER
  Top 0.305: U1.23 9.62,12.97 9.62,13.93 10.3,14.6 11.62,14.6 12.16,15.14 U8.1
C1N
  Bottom 0.305: C23.1 9.11,18.37 12.86,22.13 U$30.C1N
C1P
  Bottom 0.305: C23.2 7.63,17.04 8.51,17.04 13.56,22.1 U$30.C1P
C2N
  Bottom 0.203: C12.1
  Bottom 0.305: U$30.C2N 14.26,22 15.36,20.9 C12.1
C2P
  Bottom 0.305: C12.2 16.51,20.63 14.96,22.18 U$30.C2P
DAC  (via drill 0.25)
  Top 0.203: v16.76,7.41 16.32,7.41 16,7.73 U1.3
  Bottom 0.254: R21.1 17.98,7.41 v16.76,7.41
EN_DCDC  (via drill 0.25)
  Top 0.203: U1.25 8.41,12.77 7.56,13.62 v7.56,13.64 | v17.02,26.49 17.34,26.17 17.34,26.18 J1.9 J1.11
  Top 0.305: EN_DCDC.TP 7.99,13.62
  Top 0.406: 7.99,13.62 7.56,13.62
  Route2 0.203: v7.56,13.64 7.56,14.46 8.94,15.84 12.69,15.84 15.1,18.26 15.1,24.09 17.02,26 v17.02,26.49
EN_VCC_2  (via drill 0.25)
  Top 0.203: U1.15 13.63,13.39 13.06,13.96 v13.06,13.97 13.06,14.63
  Top 0.305: 13.06,14.63 Q3.1 13.78,14.7 R16.2
  Bottom 0.203: 17.32,24.64 17.66,24.3 17.66,21.47 17.04,20.86 17.04,19.84 17.48,19.39 17.48,16.85
  Bottom 0.254: 17.32,24.64 17.11,24.85 Q4.1 | 17.48,16.85 17.25,16.62 13.15,16.62 12.3,15.76 12.3,14.32 12.65,13.97 v13.06,13.97
FB_DAC  (via drill 0.25, 0.35)
  Top 0.203: v19.17,25.41 18.73,24.98 J1.3 | FB_DAC.TP 18.66,20.78 v19.12,20.32
  Route2 0.203: v16.63,8.69 16.63,9.29 17.83,10.49 17.83,19.13 19.02,20.32 v19.12,20.32 19.14,20.34 19.14,25.38 v19.17,25.41
  Bottom 0.254: v16.63,8.69 17.38,8.69 17.51,8.56 19.33,8.56 19.33,8.45 19.37,8.49 R20.2 19.37,7.64 R21.2
GND  (via drill 0.25, 0.35)
  Top 0.203: U3.4 1.13,12.08 1.13,11.77 | 2.02,12.98 2.06,13.02 | C14.2 19.67,9.02 | 19.67,7.6 C4.2 | U1.42 11.63,5.1 10.3,3.77 C1.2 | R17.1 15.18,1.21 15.36,1.03 C28.2 17.2,1.03 v17.44,0.8 | 1.22,5.43 R11.2 | U1.THERMAL 12.7,9.48 13.45,8.73 | U1.THERMAL 11.86,9.46 v11.86,9.09 10,7.23 U1.35 | U1.THERMAL 11.63,9.23 | U1.THERMAL 12.13,9.73 | v2.82,19.07 2.82,19.12 | 19.36,12.4 C9.2 | 19.35,11.04 C3.2 19.49,10.77 | 4.38,10.37 C8.2 4.61,10.38 4.7,10.47 | 5.83,10.47 C7.2 | v20.08,6.05 20.08,6.08 | 19.67,6.5 19.67,6.6 | C18.2 4.66,8.35 | J1.20 14.89,28.74 v14.53,29.1 | U8.2 U8.3 | J1.8 13.99,25.77 13.69,25.46 13.78,25.38 J1.6 15.46,25.38 v15.67,25.58 15.47,25.78 J1.8
  Top 0.254: 1.13,12.08 2.02,12.98 | 2.06,13.02 2.06,14.5 U3.2 | C6.2 4.5,13.66 4.18,13.34 | 1.13,11.77 1.98,10.92 2.88,10.92 3.44,10.37 4.38,10.37 | 19.67,6.6 19.67,6.63 | 19.67,7.6 19.67,9.02 | U1.5 13.45,8.73 | 11.63,9.23 U1.42 | 12.13,9.73 U1.18 | 2.82,19.12 3.17,19.47 C26.2 3.74,18.61 R22.1 | C11.2 20.02,13.93 v20.02,13.96 | C27.2 16.31,16.82 C15.2 15.57,16.86 15.13,17.3 U8.3 | R16.1 13.11,16.14 12.99,16.02 Q3.2 | U8.2 13.11,18.1 v13.03,18.17
  Top 0.305: 2.06,13.02 2.39,13.34 4.18,13.34 | 19.49,10.77 C14.2 | C2.2 19.67,6.58 19.67,6.63 19.67,7.6 | U6.2 5.49,7.07 5.22,7.33 4.54,7.33 | v1.22,6.01 1.22,5.43 | VBUS4.TP 11.25,22.92 10.82,22.49 v10.82,21.64 | C11.2 19.36,12.4 | C9.2 19.35,11.04 | 4.7,10.47 5.83,10.47 | 20.08,6.08 19.67,6.5 | 4.66,8.35 4.54,8.23 | 13.69,25.46 v13.69,25.06 | U3.2 1.98,14.5 1.98,13.01 v1.8,12.83 | U8.2 13.11,16.14
  Top 0.406: U6.3 4.54,7.33 | 4.54,8.23 4.54,7.33 | 4.54,7.33 4.18,7.33 2.78,5.93 C19.2 1.81,5.42 v1.22,6.01
  Bottom 0.203: C17.2 2.24,4.62 1.22,5.64 | v1.22,6.01 | R3.1 | C21.2 5.04,27.03 5.03,27.04 C5.2
  Bottom 0.254: U$30.VSS 10.76,21.95 | S3.4 8.16,3.36 12.62,3.36 S3.3 | C20.2 2.9,30.31 2.87,30.28 2.78,30.28 v2.76,30.3 | C22.2 8.84,30.18 C10.2 | C29.2 3.59,17.41
  Bottom 0.305: v6.92,27.73 R3.1 | v2.82,19.07 3.59,18.3 3.59,17.41
  Bottom 0.406: v1.22,6.01 1.22,5.64 | v10.82,21.64 10.82,21.89 10.76,21.95
  other vias: 11.91,10.2 12.93,9.65 5.12,33.95 6.97,33.93 1.85,28.41 1.85,25.75 1.87,23.88 3.05,2.86 20.09,11.32 13.06,33.99
  pour Bottom (isolate 0.254): 3.11,37.4 18.17,37.4 22.89,32.68 22.89,-1.85 -2.17,-1.85 -2.17,32.12
  pour GND (isolate 0.254): -1.76,34.53 -0.76,35.53 19.96,35.53 23.12,32.37 23.12,-1.34 -1.76,-1.34
  pour Top: 9.63,11.73 14.14,11.73 14.14,7.28 9.63,7.28
  pour Bottom: 4.14,3.61 5.96,3.61 5.96,1.71 5.92,1.67 4.41,1.67 4.14,1.94
GND1
  pour Bottom: 2,23.12 3.73,23.12 3.73,21.61 2,21.61
IOSENSE  (via drill 0.25)
  Top 0.203: U1.7 15.84,9.73 16.21,10.11 v16.27,10.11 | J1.19 18.68,28.18 19.14,28.64 v19.14,29.38 19.14,30.05 IOSENSE.TP
  Route2 0.203: v16.27,10.11 15.66,10.72 15.66,11.18 16.11,11.63 16.65,11.63 16.93,11.92 16.93,21.84 18.09,23 18.09,28.33 v19.14,29.38
IREF
  Bottom 0.203: R3.2 7.14,25.52
  Bottom 0.305: 7.14,25.52 7.14,24.65 7.26,24.53 U$30.IREF
LDO_EN
  Top 0.305: U3.3 1.08,15.72 1.37,16.01 2.26,16.01 3.12,16.87 4.26,16.87 R22.2 5.57,16.9 R19.1
LOW_BATT  (via drill 0.25)
  Top 0.203: R48.1 | R18.1 6.3,2.32 | Q5.2 9.79,2.04 9.51,2.32 | v18.49,15.87 17.98,15.87 17.34,15.23 17.34,12.22 16.79,11.67 15.85,11.67 15.79,11.73 U1.11
  Top 0.254: R18.1 R48.1 | 9.51,2.32 6.3,2.32 | Q5.2 v11.76,2.04 v11.76,2.03
  Top 0.305: R18.1 6.44,2.46 U6.5
  GND 0.305: v11.76,2.03 11.9,1.89 16.3,1.89 19.21,4.8 19.21,15.15 v18.49,15.87
N$1
  Bottom 0.203: 7.32,6.29 S3.2 | R15.1 5.06,8.11
  Bottom 0.254: 7.32,6.29 5.65,4.62 C17.1 4.62,4.65 4.62,6.62 R7.2 4.94,6.94 4.94,7.99 5.06,8.11 | S3.2 S3.1
N$2
  Bottom 0.203: 9.23,11.44 S1.2 | R9.2 10.17,11.44 | R8.2 12.67,8.25 | 10.81,8.25 C13.1 10.47,8.55
  Bottom 0.254: 9.23,11.44 9.23,9 9.68,8.55 10.47,8.55 | 10.17,11.44 S1.2 | 12.67,8.25 10.81,8.25
N$3
  Bottom 0.203: R12.2 16.62,2.37 17.92,3.67 C16.1 17.98,4.06 R13.1 17.98,6.2 17.74,6.44 16.65,6.44 15.44,7.65 15.44,13.58 16.13,14.27 | 16.12,14.27 16.13,14.28
  Bottom 0.254: 17.71,14.27 16.13,14.27 16.12,14.27 | 16.13,14.28 16.15,14.28 15.29,15.14 14,15.14 S2.2
  Bottom 0.305: S2.1 19.17,14.9 18.34,14.9 17.71,14.27
N$4
  Bottom 0.203: 16.51,27.38 Q4.3 16.39,27.44 13.98,27.44 13.42,26.88 Q2.1
  Bottom 0.305: R4.2 16.98,28.43 16.51,27.96 16.51,27.38
N$5
  Top 0.203: X2.P$1 17.54,3.96 | 18.75,3.96 C2.1
  Top 0.254: U1.1 15.5,6.59 15.5,4.01 15.9,3.61 X2.P$1 | 18.75,3.96 17.54,3.96
N$6
  Top 0.305: Q3.3 10.56,15.94 10.56,17.79 R5.2 10.56,17.8 Q1.1
N$7
  Top 0.203: C4.1 17.96,7.04 17.68,6.77 17.2,6.77 | X2.P$2 17.2,6.77 | U1.2 15.9,7.23 16.37,6.77 17.2,6.77
N$10
  Top 0.203: R11.1 1.21,3.95 1.53,4.26 | 3.54,4.23 2.81,4.23 C19.1
  Top 0.254: 4.54,4.41 4.41,4.53 3.84,4.53 3.54,4.23 | 4.54,4.41 U6.4 | R10.1 5.29,5.17 4.54,4.41 | 1.53,4.26 C19.1
N$17
  Top 0.254: U8.6 12.16,20.51 11.29,20.51 L7.1
N$19
  Top 0.203: 9.46,20.52 L7.2
  Top 0.305: BZ1.1 8.11,21.88 9.46,20.52
N$22
  Top 0.203: U8.4 14.06,20.32 13.09,21.28 13.09,21.8 13.65,22.36 13.65,23.57 13.29,23.93 10.57,23.93 | BZ1.2 6.82,30.34
  Top 0.305: 6.82,30.34 8.07,30.34 9.05,29.36 9.05,25.46 10.57,23.93
OP_SWITCH  (via drill 0.25)
  Top 0.203: J1.17 16.96,27.78 | J1.15 16.96,27.38 16.96,27.57 16.96,27.58 16.96,27.78 | Q5.3 11.61,1.39 12.04,0.96 OP_SWITCH.TP | v16.96,31.44 16.96,27.78
  Top 0.254: Q5.3 v7.95,1.38
  Route2 0.203: v16.96,31.44 16.11,31.44 14.99,32.55 14.37,32.55 10.71,28.89 9.53,28.89 8.68,28.04 8.68,26.78 12.99,22.48 12.99,21.03 10.56,18.6 7.14,18.6 5.92,19.82 v5.92,20.04
  GND 0.254: v5.92,20.04 5.85,20.04 4.66,18.85 4.66,7.09 7.95,3.8 v7.95,1.38
PWM_DAC  (via drill 0.25)
  Top 0.203: U1.12 15.46,12.33 v16.28,12.33
  Bottom 0.254: v16.28,12.33 16.68,12.33 17.27,11.74 17.27,9.74 17.5,9.51 18.17,9.51 R20.1
RXI  (via drill 0.25)
  Top 0.203: J1.5 17.33,25.38 17.01,25.06 17.01,23.67 v16.93,23.59 16.28,22.94 RXI.TP | U1.38 9.63,5.32 v9.89,5.06
  Route2 0.203: v16.93,23.59 16.81,23.59 15.97,22.75 15.97,13.79 13.02,10.84 10.8,10.84 9.85,9.89 9.85,5.11 v9.89,5.06
S_DOWN  (via drill 0.25)
  Top 0.203: U1.13 14.63,13.52 14.84,13.73 14.84,14.1 v14.8,14.1
  Bottom 0.203: v14.8,14.1 14.8,7.51 16.5,5.81 16.82,5.81 R13.2
S_POWER  (via drill 0.25)
  Top 0.203: U1.30 7.91,9.73 7.3,10.34 v7.3,10.43
  Bottom 0.203: R15.2 6.48,8.52 6.48,10 6.91,10.43 v7.3,10.43
S_UP  (via drill 0.25)
  Top 0.203: U1.14 14.13,13.73 14.14,13.73 14.05,13.82 14.05,13.87 v13.95,13.97
  Bottom 0.203: v13.95,13.97 13.95,13.56 14.32,13.19 14.32,8.74 R8.1
SCL  (via drill 0.25)
  Top 0.203: U1.32 7.91,8.73 7.77,8.59 v7.26,8.59
  GND 0.203: 8.89,20 v8.54,20.35
  GND 0.254: v7.26,8.59 8.33,8.59 8.89,9.15 8.89,20
  Bottom 0.203: U$30.SCL 8.66,24.41 9.77,25.51 R1.1
  Bottom 0.254: U$30.SCL 8.66,20.25 8.54,20.38 v8.54,20.35
SDA  (via drill 0.25)
  Top 0.203: U1.31 7.49,9.23 v7.16,9.56
  GND 0.254: v7.16,9.56 7.2,9.6 7.77,9.6 8.24,10.07 8.24,19.47 v7.74,19.97
  Bottom 0.203: 7.98,23.23 U$30.SDA
  Bottom 0.254: U$30.SDA 7.96,21.37 7.74,21.14 v7.74,19.97
  Bottom 0.305: R2.1 7.98,25.14 7.98,23.23
SPARE1
  Top 0.203: J1.1 18.68,24.58 18.89,24.36 18.89,23.02
  pour Top: 18.36,23.92 19.43,23.92 19.43,22.42 18.36,22.42
SWCLK  (via drill 0.25)
  Top 0.203: U1.45 13.12,6 13.12,5.03 v13.53,4.62 | VBUS2.TP 12.95,26.58 J1.12 15.68,26.58 v15.69,26.59
  GND 0.203: v13.53,4.62 13.53,3.79 13.96,3.35 14.82,3.35 18.64,7.17 18.64,13.83 16.09,16.38 16.09,21.84 17.57,23.32 17.57,24.6 15.74,26.43 15.74,26.55 v15.69,26.59
SWDIO  (via drill 0.25)
  Top 0.203: U1.46 13.63,5.42 14.24,4.81 v14.24,3.98 | VBUS3.TP 12.12,24.91 12.76,25.55 v12.76,25.57 13.37,26.18 J1.10
  GND 0.254: v14.24,3.98 14.75,3.98 18.05,7.29 18.05,13.42 15.49,15.98 15.49,24.5 14.03,25.96 13.15,25.96 v12.76,25.57
TXO  (via drill 0.25)
  Top 0.203: U1.37 9.13,4.81 v9.06,4.73 | J1.7 16.7,25.78 16.37,25.44 | 16.37,25.44 16.29,25.36 v16.29,24.32 | 16.37,25.44 16.37,30.12 VBUS6.TP
  Route2 0.203: v16.29,24.32 15.53,23.56 15.53,13.92 13.11,11.5 10.77,11.5 9.22,9.95 9.22,4.89 v9.06,4.73
VBAT_LCD
  Bottom 0.203: 11.7,30.36 C25.1 | Q2.3 12.39,28.83 12.34,28.83 | 11.79,28.83 11.13,28.16 11.13,26.14 12.16,25.11
  Bottom 0.254: U$30.VBAT 12.16,25.11 | 11.7,30.36 11.7,29.47 12.34,28.83 11.79,28.83
VBUS  (via drill 0.25)
  Top 0.203: v12.35,2.68 12.25,2.78 9.4,2.78 8.99,3.2 8.99,3.7 8.68,4.01 R10.2 | R14.1 13.69,0.95 | v13.89,21.4 14.26,21.4 15.35,20.31 VBUS5.TP | J1.2 14.46,24.58 14.33,24.45 14.23,24.35 14.23,24.62 14.59,24.97 14.88,24.97 J1.4
  Top 0.254: 13.69,0.95 12.96,1.68 12.96,2.07 v12.35,2.68
  Top 0.305: U3.1 2.98,15.43 4.57,15.43 C6.1 4.69,15.23 R19.2 6.72,15.23 6.99,15.5 6.99,16.87 v6.48,17.38
  Top 0.406: v13.89,21.4 13.88,21.42 14.33,21.87 14.33,24.45
  Route2 0.203: v6.48,17.38 6.81,17.38 7.35,17.92 | v14.67,31.88 14.57,31.99 14.41,31.99 10.63,28.21 9.48,28.21 9.12,27.85 9.12,27.19 13.89,22.42 v13.89,21.4
  Route2 0.254: v13.89,21.4 13.89,21.09
  Route2 0.305: 13.89,21.09 10.72,17.92 7.35,17.92
  GND 0.203: v12.35,2.68 9.91,2.68 5.1,7.49 5.1,16 v6.48,17.38
  Bottom 0.203: 15.53,29.99 15.82,29.7 R4.1
  Bottom 0.254: 15.82,30.73 v14.67,31.88 | v6.48,17.38 6.24,17.14 C29.1
  Bottom 0.305: 15.53,29.99 14.19,29.99 13.25,29.05 13.25,28.32 12.78,27.85 12.1,27.85 11.69,27.44 Q2.2 | R4.1 15.82,30.73
VCC  (via drill 0.25)
  Top 0.203: U1.6 16.29,9.23 17.85,10.8 17.89,10.8 | U1.17 12.63,13.39 12.14,13.88 | U1.36 7.93,6.73 7.27,7.39 | U1.44 12.63,4.52 12.89,4.27 v12.89,4.05 | R48.2 4.19,0.91 | 12.61,31.38 VBUS.TP | 18.2,14.31 C11.1 | C3.1 17.89,10.8 | 17.89,10.8 18.19,10.8
  Top 0.254: v20.11,16.48 20.11,16.22 18.2,14.31 | 4.19,0.91 v3.65,1.44 | v13.77,33.22 13.77,32.54 12.61,31.38
  Top 0.305: 7.27,7.39 v7.27,7.73 | 12.14,13.88 v11.14,13.88 | 18.19,10.8 C9.1 C11.1 | R5.1 10.51,19.1 Q1.2 7.65,19.1 7.06,19.69 7.06,19.76 v6.88,19.94
  Top 0.406: v6.47,13.65 6.14,13.32 6.14,11.94 C7.1 6.04,11.84 C8.1 3.17,11.84 U3.5
  Bottom 0.203: v12.89,4.05 13.62,3.32 14.76,3.32 15.2,2.87 R12.1 | 11.12,13.88 v11.14,13.88
  Bottom 0.254: R7.1 5.86,6.73 6.44,7.31 6.85,7.31 v7.27,7.73 | R9.1 10.37,12.98 11.12,13.73 11.12,13.88
  pour Route2 (isolate 0.254, rank 2): -1.89,36.87 18.62,36.87 23.11,32.38 23.11,-2.04 -1.89,-2.04
VCC_2  (via drill 0.25)
  Top 0.203: 5.12,19.47 C26.1 4.9,20.04 4.67,20.27 2.38,20.27 VCC_2.TP | C18.1 6.36,8.35 6.44,8.27 | v14.11,30.77 14.17,30.77 15.55,29.4 15.55,27.78 | J1.16 15.45,27.38 15.55,27.49 15.55,27.6 15.55,27.61 15.55,27.78 | J1.18 15.55,27.78
  Top 0.254: U8.5 13.15,19.99 13.15,19.28 14.11,18.32 14.18,18.32 v14.2,18.34 | Q1.3 6.74,18.46 6.39,18.46 6.01,18.08 v5.89,18.08
  Top 0.305: C15.1 16,18.3 14.25,18.3 v14.2,18.34 | 6.44,8.27 U6.1 | C18.1 6.09,9.01 v5.78,9.31 | Q1.3 6.55,18.45 5.52,19.47 5.12,19.47
  Route2 0.203: v14.11,30.77 14.03,30.77 10.73,27.47 v9.85,27.47 9.81,27.43 9.81,27.26 14.54,22.52 14.54,18.68 v14.2,18.34 14.53,18.67 14.53,20.82 14.46,20.82 10.97,17.33 | 5.82,14.43 5.74,14.35
  Route2 0.254: v5.89,18.08 5.76,17.95 5.76,16.89 7.02,15.63
  Route2 0.305: 5.74,14.35 5.74,9.35 v5.78,9.31 | 10.97,17.33 8.72,17.33 7.02,15.63 5.82,14.43
  Bottom 0.203: R1.2 R2.2 | 9.82,27.44 v9.85,27.47 | R6.2 7.75,30.34 7.92,30.17 7.92,29.39 8.11,29.2 8.66,29.2 C10.1 8.71,28.63 8.84,28.5 10.15,28.5 10.23,28.42 10.26,28.45 | U$30.VDD 10.01,23.3 10.01,24.23 10.61,24.83 10.61,27.57 10.28,27.9 10.26,27.88 10.26,28.45 | C22.1 10.26,28.45
  Bottom 0.305: R1.2 9.82,27.44 | v9.85,27.47 10.26,27.88
VCC_OLED
  Bottom 0.203: C21.1 5.17,25.34
  Bottom 0.305: 5.17,25.34 4.95,25.56 4.1,25.56 C5.1 | C21.1 5.22,23.89 U$30.VCC
VCOMH
  Bottom 0.203: C20.1 4.48,28.16 5.87,28.16 6.04,27.99 6.04,25.01 6.56,24.49 U$30.VCOMH
VDDCORE
  Top 0.203: U1.43 12.13,4.1 C1.1
VINSENSE
  Top 0.203: U1.47 14.13,5.53 14.9,4.76 14.9,3.09 | R14.2 13.79,3.01 13.91,3.14 14.86,3.14 14.9,3.09 | C28.1 R17.2 14.9,2.47 14.9,3.09
VOUTSENSE  (via drill 0.25, 0.35)
  Top 0.203: U1.10 15.95,11.23 16.22,10.96 v16.36,10.96 | v19.11,26.59 19.09,26.58 18.7,26.98 J1.13 | VOUTSENSE.TP 17.17,19.88 v17.72,20.44
  Route2 0.203: v19.11,26.59 18.51,25.99 18.51,22.78 17.34,21.61 17.34,20.88 17.34,20.82 | v16.36,10.96 16.85,10.96 17.34,11.45 17.34,20.82 | v17.72,20.44 17.34,20.82

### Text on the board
tNames: VCC | TXO | IO_SENSE | !RESET | SWCLK | SWDIO | GND | RXI | VBUS | FB_DAC | VOUT / SENSE | EN_DCDC | OP_SWITCH
bNames: - | - | - | - | - | - | GND | BATT_CPU / rover R-1 / Nov'23 V5 | GND

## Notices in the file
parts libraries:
microbuilder: This work is placed in the public domain, and may be freely used for commercial and non-commercial work with the following conditions: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
SparkFun-PowerSymbols: Licensing: Creative Commons ShareAlike 4.0 International - https://creativecommons.org/licenses/by-sa/4.0
